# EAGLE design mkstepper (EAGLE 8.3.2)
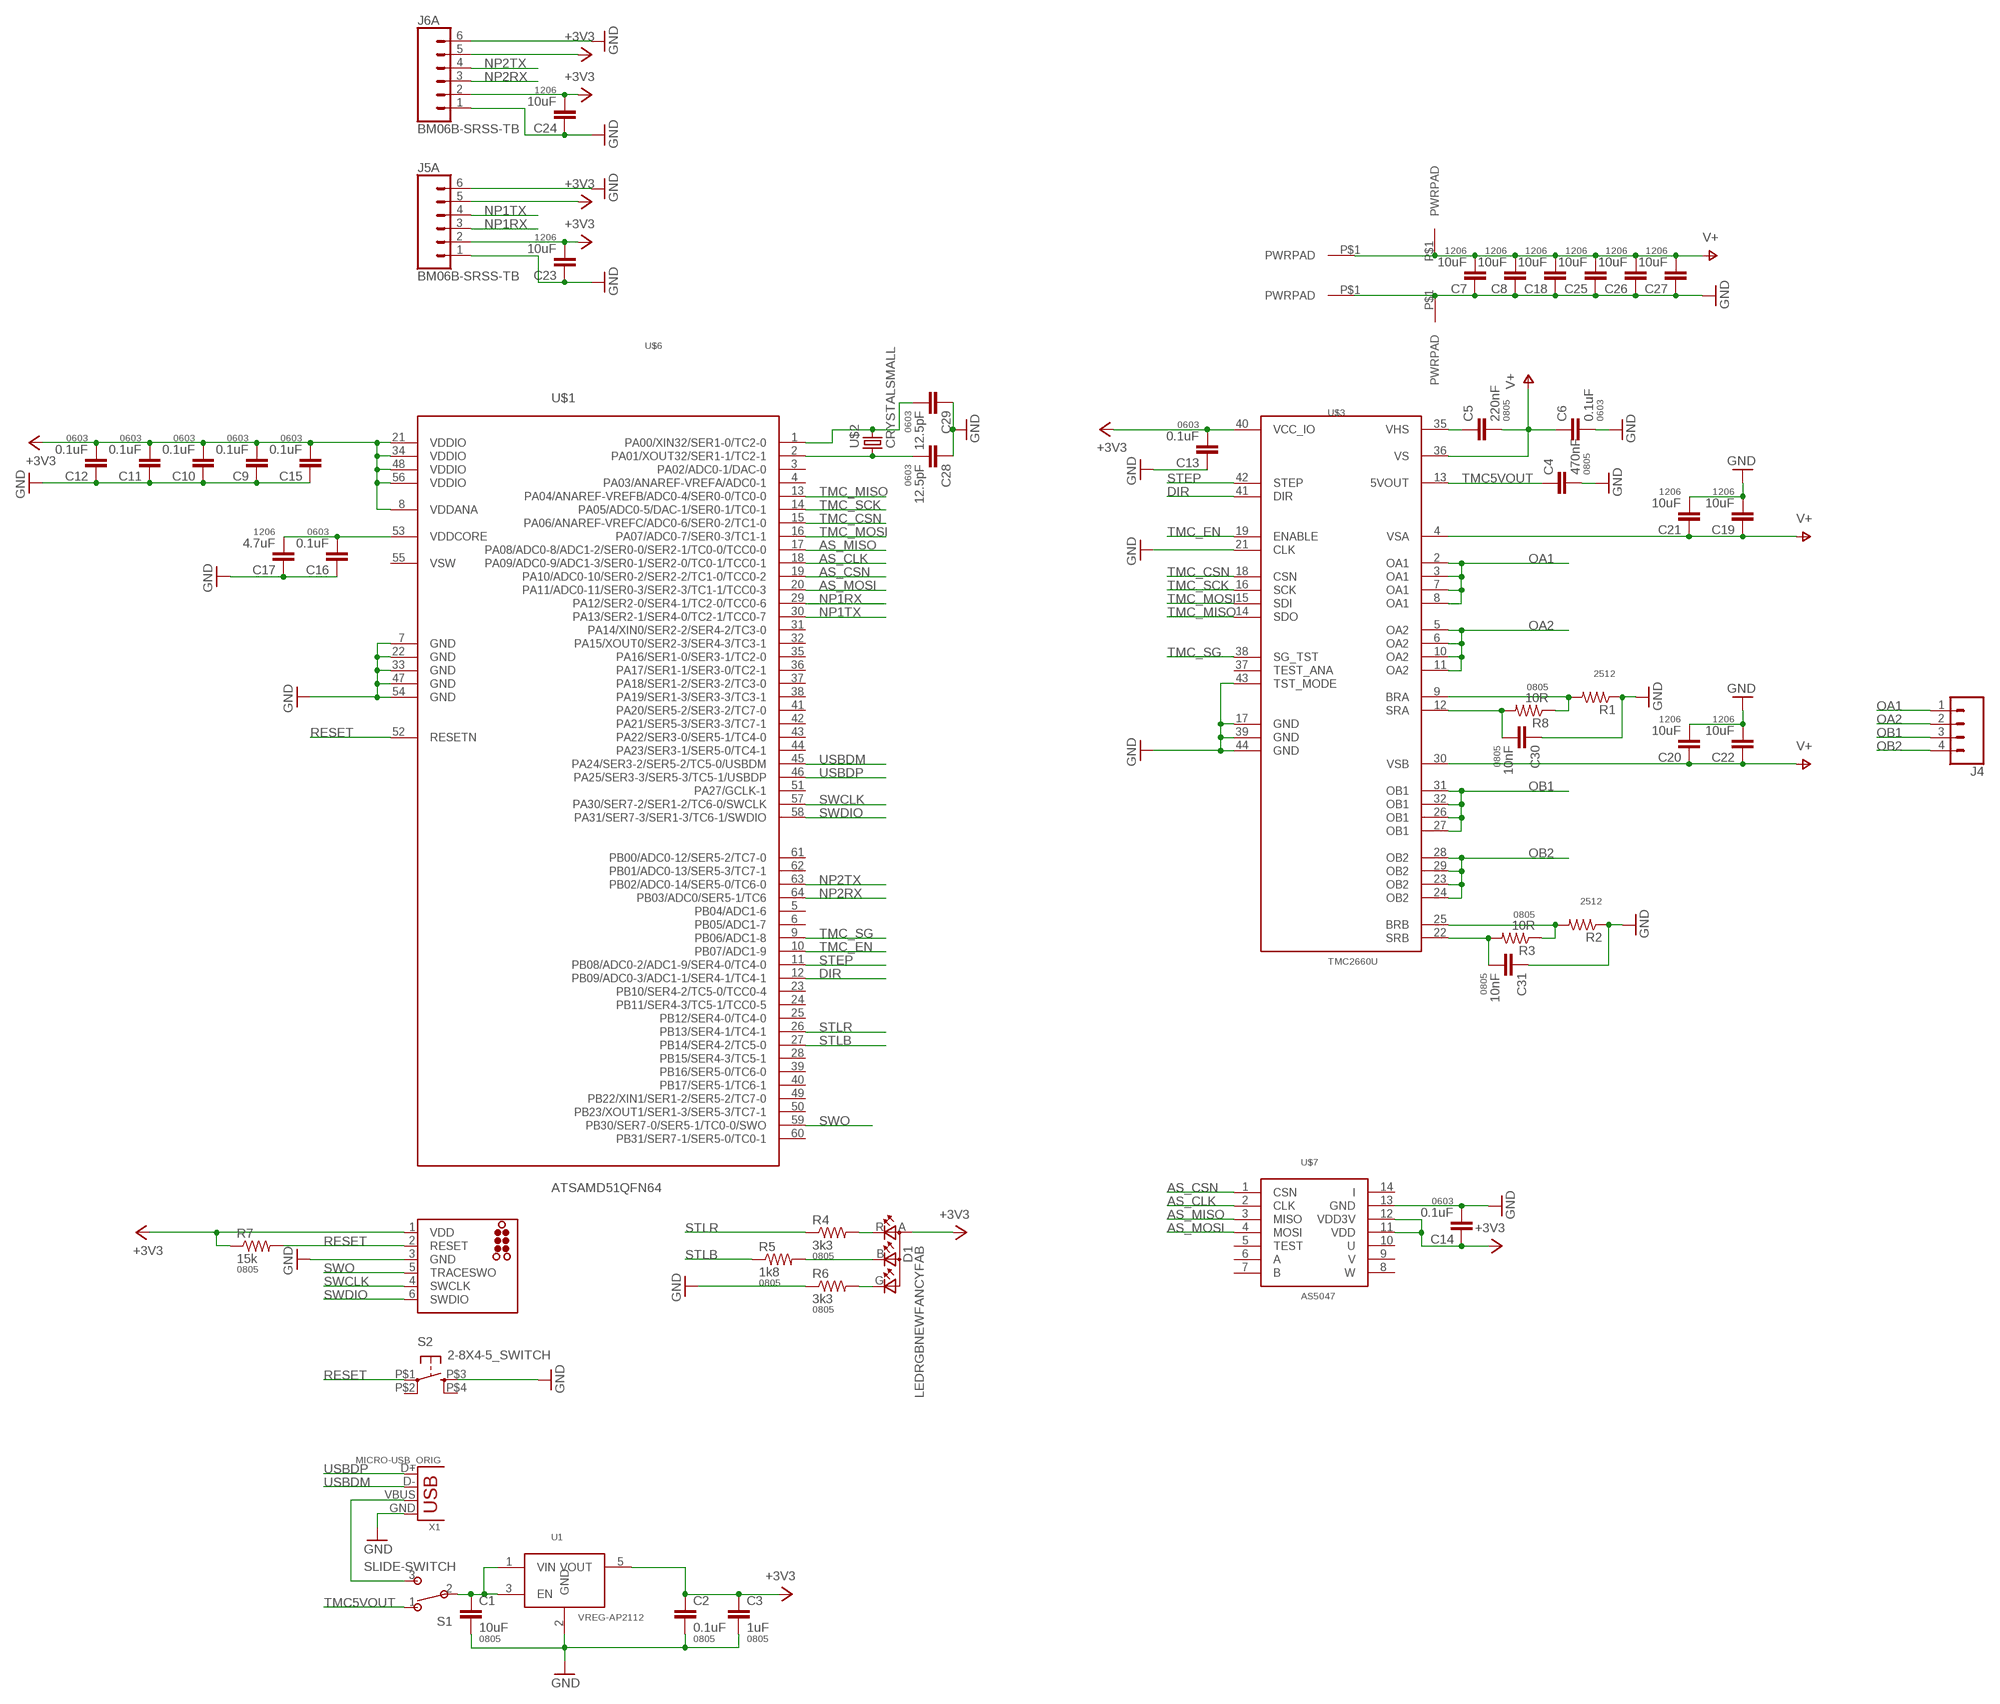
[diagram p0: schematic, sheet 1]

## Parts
C1  10uF  CAP0805  [0805]
C2  0.1uF  CAP0805  [0805]
C3  1uF  CAP0805  [0805]
C4  470nF  CAP0805  [0805]
C5  220nF  CAP0805  [0805]
C6  0.1uF  CAP0603-CAP  [0603-CAP]
C7  10uF  CAP1206  [1206]
C8  10uF  CAP1206  [1206]
C9  0.1uF  CAP0603-CAP  [0603-CAP]
C10  0.1uF  CAP0603-CAP  [0603-CAP]
C11  0.1uF  CAP0603-CAP  [0603-CAP]
C12  0.1uF  CAP0603-CAP  [0603-CAP]
C13  0.1uF  CAP0603-CAP  [0603-CAP]
C14  0.1uF  CAP0603-CAP  [0603-CAP]
C15  0.1uF  CAP0603-CAP  [0603-CAP]
C16  0.1uF  CAP0603-CAP  [0603-CAP]
C17  4.7uF  CAP1206  [1206]
C18  10uF  CAP1206  [1206]
C19  10uF  CAP1206  [1206]
C20  10uF  CAP1206  [1206]
C21  10uF  CAP1206  [1206]
C22  10uF  CAP1206  [1206]
C23  10uF  CAP1206  [1206]
C24  10uF  CAP1206  [1206]
C25  10uF  CAP1206  [1206]
C26  10uF  CAP1206  [1206]
C27  10uF  CAP1206  [1206]
C28  12.5pF  CAP0603-CAP  [0603-CAP]
C29  12.5pF  CAP0603-CAP  [0603-CAP]
C30  10nF  CAP0805  [0805]
C31  10nF  CAP0805  [0805]
D1  LEDRGBNEWFANCYFAB  [P-LCC-4-FANCYFAB]
J1  TC2030-SWD-MCP  [TC2030-MCP]
J2  PWRPADM2  [PWRPAD_2-05MM]
J3  PWRPADM2  [PWRPAD_2-05MM]
J4  CONN_04LONGPADS  [1X04_LONGPADS]
J5  BM06B-SRSS-TB  JST_6_PIN_HORIZONTAL  [JST-6-SMD-HORI-1.0MM]
J6  BM06B-SRSS-TB  JST_6_PIN_HORIZONTAL  [JST-6-SMD-HORI-1.0MM]
J7  PWRPADM2  [PWRPAD_2-05MM]
J9  PWRPADM2  [PWRPAD_2-05MM]
R1  RESISTOR2512  [R2512]
R2  RESISTOR2512  [R2512]
R3  10R  RESISTOR0805-RES  [0805]
R4  3k3  RESISTOR0805-RES  [0805]
R5  1k8  RESISTOR0805-RES  [0805]
R6  3k3  RESISTOR0805-RES  [0805]
R7  15k  RESISTOR0805-RES  [0805]
R8  10R  RESISTOR0805-RES  [0805]
S1  SLIDE-SWITCH  [AYZ0102AGRLC]
S2  2-8X4-5_SWITCH  [TACT-SWITCH-KMR6]
U1  VREG-AP2112  [SOT23-5]
U$1  ATSAMD51QFN64  [QFN-64-9X9MM]
U$2  CRYSTALSMALL  [2-SMD-1-5X3-2MM]
U$3  TMC2660U  [TQFP44]
U$6  NEMA17  [NEMA17]
U$7  AS5047  [TSSOP14]
X1  MICRO-USB_ORIG  [DX4R005HJ5]

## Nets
+3V3: C2.1 C3.1 C9.2 C10.2 C11.2 C12.2 C13.2 C14.1 C15.2 C23.2 C24.2 D1.A(A2) J1.1(VDD) J5.2 J5.5 J6.2 J6.5 R7.1 U1.5(VOUT) U$1.8(VDDANA) U$1.21(VDDIO) U$1.34(VDDIO) U$1.48(VDDIO) U$1.56(VDDIO) U$3.40(VCC_IO) U$7.11(VDD) U$7.12(VDD3V)
AS_CLK: U$1.18(PA09/ADC0-9/ADC1-3/SER0-1/SER2-0/TC0-1/TCC0-1) U$7.2(CLK)
AS_CSN: U$1.19(PA10/ADC0-10/SER0-2/SER2-2/TC1-0/TCC0-2) U$7.1(CSN)
AS_MISO: U$1.17(PA08/ADC0-8/ADC1-2/SER0-0/SER2-1/TC0-0/TCC0-0) U$7.3(MISO)
AS_MOSI: U$1.20(PA11/ADC0-11/SER0-3/SER2-3/TC1-1/TCC0-3) U$7.4(MOSI)
BRA: R1.2 R8.1 U$3.9(BRA)
BRB: R2.2 R3.1 U$3.25(BRB)
DIR: U$1.12(PB09/ADC0-3/ADC1-1/SER4-1/TC4-1) U$3.41(DIR)
GND: C1.2 C2.2 C3.2 C4.2 C6.2 C7.1 C8.1 C9.1 C10.1 C11.1 C12.1 C13.1 C14.2 C15.1 C16.1 C17.1 C18.1 C19.2 C20.2 C21.2 C22.2 C23.1 C24.1 C25.1 C26.1 C27.1 C28.1 C29.1 C30.1 C31.1 J1.3(GND) J3.P$1(PWRPAD) J5.1 J5.6 J6.1 J6.6 J7.P$1(PWRPAD) R1.1 R2.1 R6.1 S2.P$3(S) U1.2(GND) U$1.7(GND) U$1.22(GND) U$1.33(GND) U$1.47(GND) U$1.54(GND) U$3.17(GND) U$3.21(CLK) U$3.39(GND) U$3.43(TST_MODE) U$3.44(GND) U$7.13(GND) X1.GND
N$1: D1.G(CGREEN) R6.2
N$2: C5.1 U$3.35(VHS)
N$3: C1.1 S1.2 U1.1(VIN) U1.3(EN)
N$4: S1.3 X1.VBUS
N$5: D1.B(CBLUE) R5.2
N$6: D1.R(CRED) R4.2
N$7: C16.2 C17.2 U$1.53(VDDCORE)
N$8: C28.2 U$1.2(PA01/XOUT32/SER1-1/TC2-1) U$2.P$1
N$12: C29.2 U$1.1(PA00/XIN32/SER1-0/TC2-0) U$2.P$2
NP1RX: J5.3 U$1.29(PA12/SER2-0/SER4-1/TC2-0/TCC0-6)
NP1TX: J5.4 U$1.30(PA13/SER2-1/SER4-0/TC2-1/TCC0-7)
NP2RX: J6.3 U$1.64(PB03/ADC0/SER5-1/TC6)
NP2TX: J6.4 U$1.63(PB02/ADC0-14/SER5-0/TC6-0)
OA1: J4.1 U$3.2(OA1) U$3.3(OA1) U$3.7(OA1) U$3.8(OA1)
OA2: J4.2 U$3.5(OA2) U$3.6(OA2) U$3.10(OA2) U$3.11(OA2)
OB1: J4.3 U$3.26(OB1) U$3.27(OB1) U$3.31(OB1) U$3.32(OB1)
OB2: J4.4 U$3.23(OB2) U$3.24(OB2) U$3.28(OB2) U$3.29(OB2)
RESET: J1.2(RESET) R7.2 S2.P$1(P) U$1.52(RESETN)
SRA: C30.2 R8.2 U$3.12(SRA)
SRB: C31.2 R3.2 U$3.22(SRB)
STEP: U$1.11(PB08/ADC0-2/ADC1-9/SER4-0/TC4-0) U$3.42(STEP)
STLB: R5.1 U$1.27(PB14/SER4-2/TC5-0)
STLR: R4.1 U$1.26(PB13/SER4-1/TC4-1)
SWCLK: J1.4(SWCLK) U$1.57(PA30/SER7-2/SER1-2/TC6-0/SWCLK)
SWDIO: J1.6(SWDIO) U$1.58(PA31/SER7-3/SER1-3/TC6-1/SWDIO)
SWO: J1.5(TRACESWO) U$1.59(PB30/SER7-0/SER5-1/TC0-0/SWO)
TMC5VOUT: C4.1 S1.1 U$3.13(5VOUT)
TMC_CSN: U$1.15(PA06/ANAREF-VREFC/ADC0-6/SER0-2/TC1-0) U$3.18(CSN)
TMC_EN: U$1.10(PB07/ADC1-9) U$3.19(ENABLE)
TMC_MISO: U$1.13(PA04/ANAREF-VREFB/ADC0-4/SER0-0/TC0-0) U$3.14(SDO)
TMC_MOSI: U$1.16(PA07/ADC0-7/SER0-3/TC1-1) U$3.15(SDI)
TMC_SCK: U$1.14(PA05/ADC0-5/DAC-1/SER0-1/TC0-1) U$3.16(SCK)
TMC_SG: U$1.9(PB06/ADC1-8) U$3.38(SG_TST)
USBDM: U$1.45(PA24/SER3-2/SER5-2/TC5-0/USBDM) X1.D-
USBDP: U$1.46(PA25/SER3-3/SER5-3/TC5-1/USBDP) X1.D+
V+: C5.2 C6.1 C7.2 C8.2 C18.2 C19.1 C20.1 C21.1 C22.1 C25.2 C26.2 C27.2 J2.P$1(PWRPAD) J9.P$1(PWRPAD) U$3.4(VSA) U$3.30(VSB) U$3.36(VS)
Unconnected: J5.M1 J5.M2 J6.M1 J6.M2 S2.P$2(P1) S2.P$4(S1) U$1.3(PA02/ADC0-1/DAC-0) U$1.4(PA03/ANAREF-VREFA/ADC0-1) U$1.5(PB04/ADC1-6) U$1.6(PB05/ADC1-7) U$1.23(PB10/SER4-2/TC5-0/TCC0-4) U$1.24(PB11/SER4-3/TC5-1/TCC0-5) U$1.25(PB12/SER4-0/TC4-0) U$1.28(PB15/SER4-3/TC5-1) U$1.31(PA14/XIN0/SER2-2/SER4-2/TC3-0) U$1.32(PA15/XOUT0/SER2-3/SER4-3/TC3-1) U$1.35(PA16/SER1-0/SER3-1/TC2-0) U$1.36(PA17/SER1-1/SER3-0/TC2-1) U$1.37(PA18/SER1-2/SER3-2/TC3-0) U$1.38(PA19/SER1-3/SER3-3/TC3-1) U$1.39(PB16/SER5-0/TC6-0) U$1.40(PB17/SER5-1/TC6-1) U$1.41(PA20/SER5-2/SER3-2/TC7-0) U$1.42(PA21/SER5-3/SER3-3/TC7-1) U$1.43(PA22/SER3-0/SER5-1/TC4-0) U$1.44(PA23/SER3-1/SER5-0/TC4-1) U$1.49(PB22/XIN1/SER1-2/SER5-2/TC7-0) U$1.50(PB23/XOUT1/SER1-3/SER5-3/TC7-1) U$1.51(PA27/GCLK-1) U$1.55(VSW) U$1.60(PB31/SER7-1/SER5-0/TC0-1) U$1.61(PB00/ADC0-12/SER5-2/TC7-0) U$1.62(PB01/ADC0-13/SER5-3/TC7-1) U$3.37(TEST_ANA) U$7.5(TEST) U$7.6(A) U$7.7(B) U$7.8(W) U$7.9(V) U$7.10(U) U$7.14(I)

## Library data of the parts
C1-C5 C30 C31 = borkedlabs-passives:CAP: Capacitor; PACKAGE: 0805
C6 C9-C16 C28 C29 = borkedlabs-passives:CAP: Capacitor; PACKAGE: 0603
C7 C8 C17-C27 = borkedlabs-passives:CAP: Capacitor; PACKAGE: 1206
D1 = fab:LEDRGBNEW
J1 = atsam:TC2030-SWD: TAG-CONNECT ICSP Connector Manufacturer: Tag-Connect Cable for easy In-Circuit Serial Programming. Designed for Microchip ICD2, suitable for many others. Two variants - one "with legs" (for hands-free fit on PCB) and another "without legs" for quick programming. PADDescription 1MCLR/Vpp 2Vdd 3GND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
J2 J3 J7 J9 = power:PWRPAD
J4 = SparkFun-Connectors:CONN_04: Multi connection point. Often used as Generic Header-pin footprint for 0.1 inch spaced/style header connections On any of the 0.1 inch spaced packages, you can populate with these: Break Away Headers - Straight (PRT-00116) Break Away Male Headers - Right Angle (PRT-00553) Female Headers (PRT-00115)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; PROD_ID: CONN-09696
J5 J6 = SparkFun-Connectors:JST_6_PIN_HORIZONTAL: JST 6 pin horizontal connector JST-SH type. Here is the connector we sell at SparkFun: name (XXX-00000) Datasheet It was used on these SparkFun products: name (XXX-00000) name (XXX-00000); PROD_ID: XXX-00000
R1 R2 = borkedlabs-passives:RESISTOR: Resistor; PACKAGE: 2512
R3-R8 = borkedlabs-passives:RESISTOR: Resistor; PACKAGE: 0805
S1 = fab:SLIDE-SWITCH: SMD slide-switch AYZ0102AGRLC as found in the fablab inventory. Includes the mounting holes. Made by Zaerc.
S2 = fab:2-8X4-5_SWITCH
U1 = power:VREG-AP2112
U$1 = atsam:ATSAMD51
U$2 = fab:CRYSTAL
U$3 = power:TMC2660
U$6 = motors:NEMA17
U$7 = sensor:AS5047
X1 = fab:MICRO-USB: SMD micro USB connector as found in the fablab inventory. Three footprint variants included: original, as described by manufacturer's datasheet for milling with the 1/100" bit for milling with the 1/64" bit Made by Zaerc.

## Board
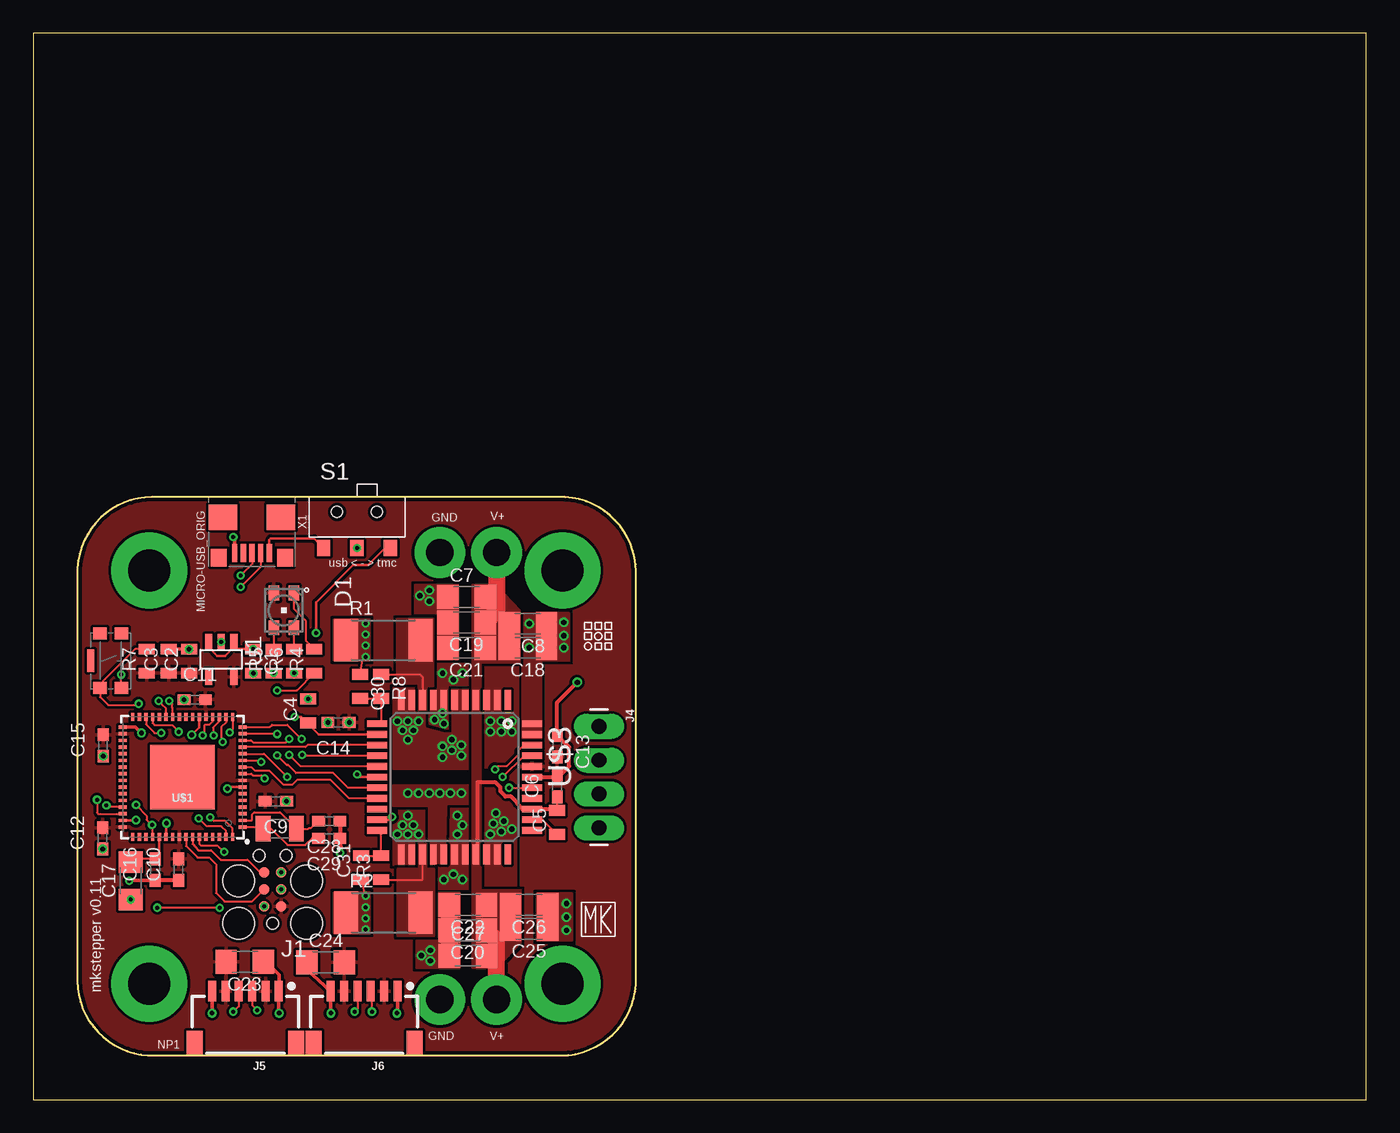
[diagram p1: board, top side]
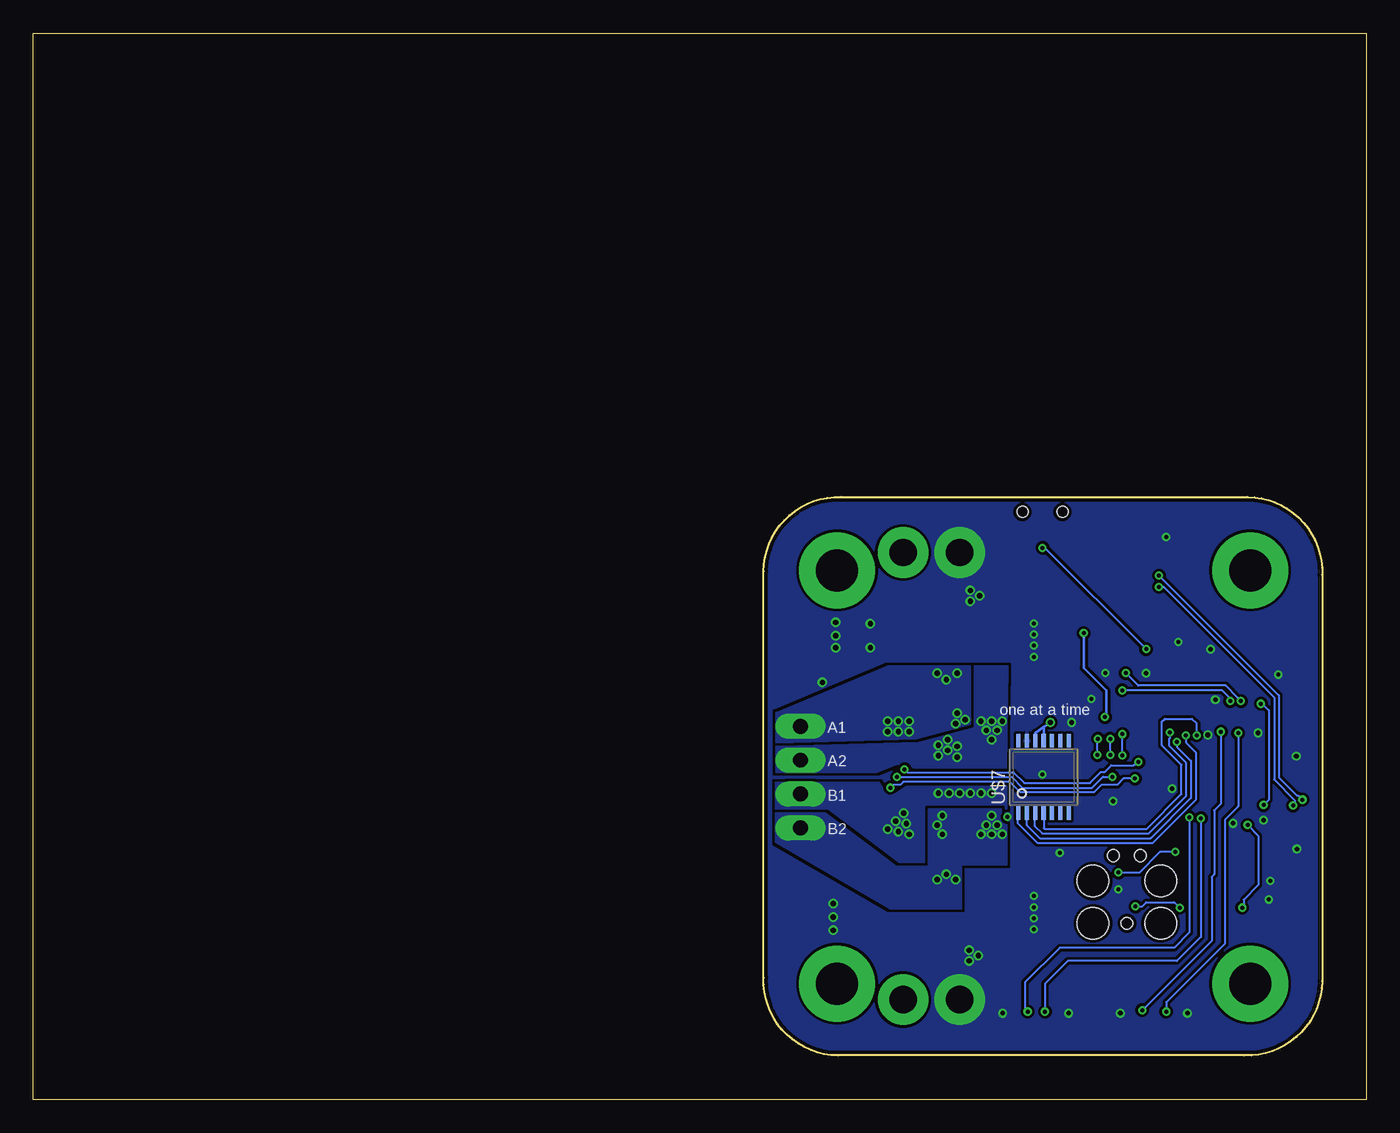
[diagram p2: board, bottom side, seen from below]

Size 100 x 80 mm. Coordinates in mm from the lower left corner, seen from the top.
Outline: 0,0 100,0 100,80 0,80 0,0
Outline: 8.89,45.21 arc91 3.3,39.37 3.3,8.89 arc91 9.14,3.3 39.62,3.3 arc91 45.21,9.14 45.21,39.62 arc91 39.37,45.21 8.89,45.21
Copper layers (1*16): Top 0.035mm / dielectric 1.5mm / Bottom 0.035mm
Design rules "default *": minimum track width 6mil, minimum drill 0.3mm, track to track 8mil, track to pad 8mil, pad to pad 8mil, via to via 8mil, smd to smd 8mil, copper to edge 10mil, drill to drill 10mil, minimum pad ring 6mil, minimum via ring 6mil, stop-mask expansion 4mil, vias tented up to drill 27mil, thermal gap 9mil

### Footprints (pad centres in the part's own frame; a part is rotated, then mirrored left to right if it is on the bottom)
0805 = smd 0.8 x 1.2: 1 -0.9,0; 2 0.9,0
0603-CAP = smd 0.96 x 0.8: 1 -0.8,0; 2 0.8,0
1206 = smd 1.6 x 1.8: 1 -1.4,0; 2 1.4,0
P-LCC-4-FANCYFAB = smd 0.8 x 1.1: A 0.75,-1.3; B 0.75,1.3; G -0.75,1.3; R -0.75,-1.3
TC2030-MCP = smd 0.787 x 0.787: 1 1.27,-0.635; 2 1.27,0.635; 3 2.54,-0.635; 4 2.54,0.635; 5 3.81,-0.635; 6 3.81,0.635 | hole 0.889: 0,0; 5.08,-1.016; 5.08,1.016 | hole 2.375: 0,2.54; 0,-2.54; 3.175,-2.54; 3.175,2.54
PWRPAD_2-05MM = drill 2.05 pad 3.8: P$1 0,0
1X04_LONGPADS = drill 1.118 pad 1.88 long: 1 0,0; 2 2.54,0; 3 5.08,0; 4 7.62,0
JST-6-SMD-HORI-1.0MM = smd 0.6 x 1.55: 1 -2.5,-4.775; 2 -1.5,-4.775; 3 -0.5,-4.775; 4 0.5,-4.775; 5 1.5,-4.775; 6 2.5,-4.775 | smd 1.2 x 1.8: M1 -3.8,-0.9; M2 3.8,-0.9
R2512 = smd 1.8 x 3.2: 1 -2.8,0; 2 2.8,0
AYZ0102AGRLC = smd 1 x 1.2: 1 2.5,-2.3; 2 0,-2.3; 3 -2.5,-2.3 | hole 0.85: -1.5,0.4; 1.5,0.4
TACT-SWITCH-KMR6 = smd 0.9 x 1: P$1 -2.05,0.8; P$2 2.05,0.8; P$3 -2.05,-0.8; P$4 2.05,-0.8 | smd 1.7 x 0.55: P$5 0,1.5
SOT23-5 = smd 0.533 x 1.194: 1 -0.95,-1.306; 2 0,-1.306; 3 0.95,-1.306; 4 0.95,1.306; 5 -0.95,1.306
QFN-64-9X9MM = smd 0.6 x 0.25: 1 -4.5,3.75; 2 -4.5,3.25; 3 -4.5,2.75; 4 -4.5,2.25; 5 -4.5,1.75; 6 -4.5,1.25; 7 -4.5,0.75; 8 -4.5,0.25; 9 -4.5,-0.25; 10 -4.5,-0.75; 11 -4.5,-1.25; 12 -4.5,-1.75; 13 -4.5,-2.25; 14 -4.5,-2.75; 15 -4.5,-3.25; 16 -4.5,-3.75; 33 4.5,-3.75; 34 4.5,-3.25; 35 4.5,-2.75; 36 4.5,-2.25; 37 4.5,-1.75; 38 4.5,-1.25; 39 4.5,-0.75; 40 4.5,-0.25; 41 4.5,0.25; 42 4.5,0.75; 43 4.5,1.25; 44 4.5,1.75; 45 4.5,2.25; 46 4.5,2.75; 47 4.5,3.25; 48 4.5,3.75 | smd 0.25 x 0.6: 17 -3.75,-4.5; 18 -3.25,-4.5; 19 -2.75,-4.5; 20 -2.25,-4.5; 21 -1.75,-4.5; 22 -1.25,-4.5; 23 -0.75,-4.5; 24 -0.25,-4.5; 25 0.25,-4.5; 26 0.75,-4.5; 27 1.25,-4.5; 28 1.75,-4.5; 29 2.25,-4.5; 30 2.75,-4.5; 31 3.25,-4.5; 32 3.75,-4.5; 49 3.75,4.5; 50 3.25,4.5; 51 2.75,4.5; 52 2.25,4.5; 53 1.75,4.5; 54 1.25,4.5; 55 0.75,4.5; 56 0.25,4.5; 57 -0.25,4.5; 58 -0.75,4.5; 59 -1.25,4.5; 60 -1.75,4.5; 61 -2.25,4.5; 62 -2.75,4.5; 63 -3.25,4.5; 64 -3.75,4.5 | smd 4.826 x 4.826: P$1 0,0
2-SMD-1-5X3-2MM = smd 1.1 x 1.9: P$1 -1.25,0; P$2 1.25,0
TQFP44 = smd 1.5 x 0.5: 1 -5.8,4; 2 -5.8,3.2; 3 -5.8,2.4; 4 -5.8,1.6; 5 -5.8,0.8; 6 -5.8,0; 7 -5.8,-0.8; 8 -5.8,-1.6; 9 -5.8,-2.4; 10 -5.8,-3.2; 11 -5.8,-4; 23 5.8,-4; 24 5.8,-3.2; 25 5.8,-2.4; 26 5.8,-1.6; 27 5.8,-0.8; 28 5.8,0; 29 5.8,0.8; 30 5.8,1.6; 31 5.8,2.4; 32 5.8,3.2; 33 5.8,4 | smd 0.5 x 1.5: 12 -4,-5.8; 13 -3.2,-5.8; 14 -2.4,-5.8; 15 -1.6,-5.8; 16 -0.8,-5.8; 17 0,-5.8; 18 0.8,-5.8; 19 1.6,-5.8; 20 2.4,-5.8; 21 3.2,-5.8; 22 4,-5.8; 34 4,5.8; 35 3.2,5.8; 36 2.4,5.8; 37 1.6,5.8; 38 0.8,5.8; 39 0,5.8; 40 -0.8,5.8; 41 -1.6,5.8; 42 -2.4,5.8; 43 -3.2,5.8; 44 -4,5.8
NEMA17 = drill 3.15 pad 5.7: P$1 -15.5,15.5; P$2 15.5,15.5; P$3 -15.5,-15.5; P$4 15.5,-15.5
TSSOP14 = smd 0.305 x 0.991: 1 -1.905,-2.718; 2 -1.27,-2.718; 3 -0.635,-2.718; 4 0,-2.718; 5 0.635,-2.718; 6 1.27,-2.718; 7 1.905,-2.718; 8 1.905,2.718; 9 1.27,2.718; 10 0.635,2.718; 11 0,2.718; 12 -0.635,2.718; 13 -1.27,2.718; 14 -1.905,2.718
DX4R005HJ5 = smd 0.4 x 1.35: D+ 0,1.6; D- -0.65,1.6; GND 1.3,1.6; ID 0.65,1.6; VBUS -1.3,1.6 | smd 1.2 x 1.3: GND@1 -2.5,1.95; GND@2 2.5,1.95 | smd 2.15 x 1.9: GND@3 -2.175,-1.1; GND@4 2.175,-1.1

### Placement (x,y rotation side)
C1  16.51,32.89 270 top
C2  11.68,32.89 90 top
C3  10.16,32.89 90 top
C4  20.61,29.16 90 top
C5  39.3,20.8 90 top
C6  39.3,23.5 90 top
C7  32.5,37.7 0 top
C8  37.1,35.7 180 top
C9  18.2,22.38 180 top
C10  10.9,17.25 90 top
C11  12.11,30 0 top
C12  5.2,19.6 90 top
C13  39.3,26.5 270 top
C14  22.9,28.3 180 top
C15  5.24,26.57 90 top
C16  9.15,17.25 90 top
C17  7.3,16.4 90 top
C18  37.1,33.9 180 top
C19  32.5,35.8 180 top
C20  32.6,12.7 180 top
C21  32.5,33.9 180 top
C22  32.6,14.6 180 top
C23  15.87,10.32 180 top
C24  21.93,10.3 0 top
C25  37.2,12.8 180 top
C26  37.2,14.6 180 top
C27  32.6,10.8 0 top
C28  22.2,20.9 180 top
C29  22.2,19.6 180 top
C30  24.5,31 270 top
C31  24.6,17.4 90 top
D1  18.8,36.7 180 top
J1  17.95,13.22 90 top
J2  34.75,41.04 0 top
J3  30.5,41.04 0 top
J4  42.45,28 270 top
J5  15.92,3.35 180 top
J6  24.82,3.35 180 top
J7  30.5,7.5 0 top
J9  34.75,7.5 0 top
R1  26.26,34.47 0 top
R2  26.27,14.01 0 top
R3  26.1,17.4 90 top
R4  21.08,32.89 90 top
R5  18.03,32.89 90 top
R6  19.56,32.89 90 top
R7  8.51,32.89 90 top
R8  26.1,31 270 top
S1  24.28,43.69 0 top
S2  5.81,32.92 90 top
U1  14.1,33.02 180 top
U$1  11.2,24.2 180 top
U$2  18.49,20.32 180 top
U$3  31.6,24.2 270 top
U$5  [CBA-SILK-LOGO]  42.38,34.77 90 top
U$6  24.2,24.2 0 top
U$7  24.2,24.2 0 bottom
U$9  [MK-LOGO-SILK]  42.38,13.51 0 top
X1  16.4,42.6 180 top

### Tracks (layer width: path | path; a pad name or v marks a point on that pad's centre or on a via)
+3V3  (via drill 0.35)
  Bottom 0.2: C14.1 23.9,28.15 24.13,28 | U$7.12 24.84,27.52 24.13,28 | U$7.11 24.2,27.92 24.13,28
  other vias: 23.7,28.3
  pour Top (rank 6): 3.15,39.65 3.3,45.21 8.7,45.2 39.7,45.2 45.21,45.21 45.25,39.65 45.25,8.7 45.21,3.3 39.7,3.15 8.7,3.15 3.3,3.3 3.15,8.7
AS_CLK  (via drill 0.3 pad 0.42)
  Top 0.152: U$1.18 14.45,28.29 14.1,27.94 14.1,27.56 14.11,27.55 14.11,26.91 v14.19,26.83
  Bottom 0.152: U$7.2 25.45,21.46 25.45,20.57 24.49,19.61 16.16,19.61 13.14,22.63 13.14,25.41 14.19,26.46 v14.19,26.83
AS_CSN  (via drill 0.3 pad 0.42)
  Top 0.152: U$1.19 13.95,28.38 13.49,27.91 13.49,27.35 v13.53,27.3
  Bottom 0.152: U$7.1 26.14,21.45 26.14,20.73 24.66,19.25 16.01,19.25 12.79,22.48 12.79,26.05 13.53,26.79 v13.53,27.3
AS_MISO  (via drill 0.3 pad 0.42)
  Top 0.152: U$1.17 14.95,27.78 v14.73,27.56
  Bottom 0.152: U$7.3 24.84,20.5 24.31,19.96 16.31,19.96 13.5,22.77 13.5,25.26 14.78,26.54 14.78,27.07 14.73,27.11 v14.73,27.56
AS_MOSI  (via drill 0.3 pad 0.42)
  Top 0.152: U$1.20 13.45,28.38 13.19,28.12 12.88,28.12 12.83,28.07 12.83,27.44 v12.72,27.33
  Bottom 0.152: U$7.4 24.2,20.36 24.16,20.32 16.45,20.32 13.85,22.92 13.85,25.12 15.31,26.58 15.31,28.37 15.11,28.57 13.08,28.57 12.72,28.21 v12.72,27.33
BRA
  Top 0.152: R8.1 29,31.9 29.2,31.7 U$3.9
  pour Top (no thermals): 28.9,29.2 28.9,31.2 27.3,31.2 27.3,36.1 30,36.1 30,31 29.5,31 29.5,29.2
BRB
  Top 0.152: R3.1 29.2,16.5 U$3.25
  pour Top (no thermals): 28.9,19.2 28.9,17.3 27.3,17.3 27.3,12.3 30.1,12.3 30.1,17.3 29.5,17.3 29.5,19.2
DIR  (via drill 0.3, 0.3 pad 0.42)
  Top 0.152: U$1.12 17.31,25.95 v19.04,24.22 | U$3.41 36.8,25.8 v35.2,24.2
  Top 0.2: 36.77,25.8 U$3.41
  Bottom 0.152: v35.2,24.2 26.6,24.2 25.8,23.4 20.57,23.4 19.75,24.22 v19.04,24.22 | v19.04,24.22
GND  (via drill 0.3, 0.3 pad 0.42, 0.35, 0.4 pad 0.42)
  Top 0.152: S2.P$3 v6.61,31.87 v6.6,31.88 | v24.94,15.27 25,15.33 24.8,15.53 C31.1 | 25,33.16 v24.94,33.22 24.7,32.98 C30.1
  Top 0.2: U$3.17 24.5,24.2 v24.3,24.4 | U$3.21 26.71,21 v26.91,21.19 | 39.25,27.4 C13.1 | 39.2,24.3 C6.2
  Top 0.203: 9.09,16.34 C16.1 | U$1.54 9.95,20.69 v9.98,20.73 | U$1.47 v7.69,20.95 v7.7,20.95 | U$1.7 14.69,23.45 v14.55,23.32 | U$1.22 12.45,27.92 v11.89,27.36
  Top 0.254: X1.GND 15.1,42.13 v15.01,42.22 | U$1.33 7.66,27.95 v8.1,27.51 | C3.2 C2.2 | v18.44,6.48 18.42,6.49 J5.1 18.44,7.94 18.44,9.37 17.59,10.22 C23.1 | J5.6 13.42,6.49 v13.41,6.48 | v22.33,6.48 22.32,6.49 J6.6 20.53,9.72 C24.1 | J6.1 27.32,6.52 v27.28,6.48
  Top 0.305: C28.1 C29.1 23.05,18.55 v23,18.5 | C6.2 39.6,24.4 40.16,24.95 40.16,24.96 40.2,25 40.2,26.45 C13.1 39.3,29.8 v40.8,31.3 | U$3.39 39.1,24.2 39.2,24.3 | C10.1 C16.1 v7.2,16.4
  Top 1.27: C22.2 C20.2 C27.1 | C18.1 C8.1 | C25.1 C26.1
  other vias: 22.1,28.3 24.94,35.73 24.94,34.06 24.94,34.9 24.94,12.75 24.94,13.59 24.94,14.43 7.3,15 5.24,25.77 11.31,30 19,22.38 16.51,31.99 11.68,33.79 5.2,18.8 14.1,34.33 18.59,15.76 19.56,31.99 20.61,30.06 40,14.7 40,13.7 40,12.7 29.8,11.2 29.8,10.4 29.1,10.8 39.8,35.8 39.8,34.8 39.8,33.9 29.7,38.2 29.7,37.4 29,37.8 37.2,33.9 37.2,35.7
  pour Bottom (rank 4): 3.15,39.65 3.3,45.21 8.7,45.2 39.7,45.2 45.21,45.21 45.25,39.65 45.25,8.7 45.21,3.3 39.7,3.15 8.7,3.15 3.3,3.3 3.15,8.7
  pour Top (no thermals): 22.57,36.04 25.24,36.04 25.24,32.91 22.57,32.91
  pour Top (no thermals): 22.57,15.57 25.24,15.57 25.24,12.45 22.57,12.45
  pour Top (no thermals): 37.8,15.5 40.4,15.5 40.4,11.9 37.8,11.9
  pour Top (rank 3, no thermals): 32,9.9 32,15.5 30.4,15.5 30.4,11.9 28.7,11.9 28.7,9.9
  pour Top (no thermals): 37.7,36.5 37.7,33 40.2,33 40.2,36.5
  pour Top (rank 3, no thermals): 30.3,33 31.9,33 31.9,38.6 28.6,38.6 28.6,36.5 30.3,36.5
  pour Top (rank 2, no thermals): 36.7,27.1 36.7,36.5 40.2,36.5 40.2,32.9 38.1,32.9 38.1,27.1
N$1
  Top 0.152: D1.G 19.55,33.8 R6.2
N$2
  Top 0.2: U$3.35 38.2,21 C5.1
N$3  (via drill 0.3 pad 0.42)
  Top 0.2: U1.3 13.15,33.95 13.8,33.3 14.4,33.3 15.05,33.95 15.05,34 | 15.05,34 U1.1 | C1.1 15.25,33.79 15.05,34
  Bottom 0.2: S1.2 24.11,41.39 C1.1
  other vias: 16.51,33.79 24.28,41.39
N$4
  Top 0.2: X1.VBUS 17.7,42 17.8,42.1 21.07,42.1 S1.3
N$5
  Top 0.152: D1.B 18.05,33.8 R5.2
N$6
  Top 0.152: D1.R 19.55,36.84 20.45,35.94 20.45,34.43 R4.2
N$7
  Top 0.203: U$1.53 9.45,18.4 C16.2 7.6,18.1 C17.2
N$8
  Top 0.152: U$1.2 16.41,20.95 16.41,21.39 16.57,21.55 18.51,21.55 U$2.P$1 20.62,20.32 20.68,20.38 20.83,20.38 C28.2
N$12
  Top 0.152: U$1.1 16.91,20.45 U$2.P$2 17.84,20.32 19.07,19.09 20.4,19.09 20.91,19.6 C29.2
NP1RX  (via drill 0.3 pad 0.42)
  Top 0.152: U$1.29 8.95,28.25 9.1,28.1 10.4,28.1 v10.9,27.6 | J5.3 16.42,7.08 v16.8,6.7
  Bottom 0.152: v10.9,27.6 10.9,22.2 11.4,21.7 11.4,16.9 11.6,16.7 11.6,11.9 v16.8,6.7
NP1TX  (via drill 0.3 pad 0.42)
  Top 0.152: U$1.30 8.45,28.15 9.1,27.5 v9.6,27.5 | J5.4 15.42,6.98 v15,6.6
  Bottom 0.152: v9.6,27.5 9.6,22 10.6,21 10.6,11.7 15,7.3 v15,6.6
NP2RX  (via drill 0.3 pad 0.42)
  Top 0.152: U$1.64 14.95,20.35 14.4,20.9 13.54,20.9 v13.27,21.17 | v25.4,6.6 25.4,8.05 J6.3
  Bottom 0.152: v13.27,21.17 13.27,12.53 14.4,11.4 23,11.4 25.6,8.8 25.6,6.8 v25.4,6.6
NP2TX  (via drill 0.3 pad 0.42)
  Top 0.152: U$1.63 14.45,20.15 14.1,20.5 13,20.5 v12.4,21.1 | J6.4 24.32,6.82 v24.1,6.6
  Bottom 0.152: v12.4,21.1 12.4,12.2 14.2,10.4 22.4,10.4 24.1,8.7 v24.1,6.6
OA1  (via drill 0.4 pad 0.42)
  other vias: 30.7,29 30.8,28.2 30.1,28.5 34.3,27.6 35.1,27.6 35.9,27.6 30.7,32 32.2,32 31.5,31.5 34.3,28.4 35.1,28.4 35.9,28.4
  pour Bottom (rank 2, no thermals): 44.3,26.8 33.8,27.1 29.7,28.2 29.7,32.5 35.9,32.5 44.2,29 44.3,29
  pour Top (rank 2, no thermals): 30.2,32.7 30.2,30.9 29.7,30.9 29.7,28.2 31.1,27.8 31.1,31.1 32.8,31.1 32.8,32.7
  pour Top (rank 2, no thermals): 33.6,32.7 33.6,27.2 33.7,24.9 36.4,25 36.4,32.7
OA2  (via drill 0.4 pad 0.42)
  other vias: 28.5,27.7 28.1,28.4 28.9,28.4 27.7,27.7 27.3,28.4 28.1,27 31.4,27 31.4,26.2 32.1,26.6 32.1,25.8 30.7,26.5 30.7,25.7
  pour Bottom (rank 3, no thermals): 44.3,24.6 36.7,24.6 35.2,25.2 34.3,25.2 33.8,24.8 27,24.8 26.9,32.5 29.4,32.5 29.5,28 33.9,26.9 44.3,26.5
  pour Top (rank 3, no thermals): 28.8,30.9 27,30.9 27,24.8 33.8,24.8 34.3,25.2 35.4,25.2 36.2,26 36.2,26.8 34.3,26.8 33.5,27 33.5,29.1 32.8,29.1 32.8,30.8 31.3,30.8 31.3,27.6 29.5,28.1 29.5,29.1 28.8,29.1
OB1  (via drill 0.4 pad 0.42)
  other vias: 29.7,23 28.9,23 28.1,23 30.5,23 31.3,23 32.1,23 34.3,19.9 35.1,20.1 34.7,21.5 35.9,20.3 35.3,20.9 34.5,20.7
  pour Bottom (rank 2, no thermals): 44.3,23.8 36.6,23.8 36.1,23 36,22.9 35.4,22.9 34.3,23.6 27,23.6 27,21.8 32.9,21.8 32.9,17.7 35.2,17.7 36.3,18.6 40.8,21.8 44.3,21.8
  pour Top (rank 4, no thermals): 29.7,17.6 29.7,22 27,22 27,23.6 34.3,23.6 35.4,22.9 36.2,22.9 36.2,15.8 33.6,15.8 33.6,19.4 32.9,19.4 33,21.8 31.2,21.8 31.1,17.6
OB2  (via drill 0.4 pad 0.42)
  other vias: 28.1,19.9 27.3,19.9 28.9,19.9 27.7,20.6 28.5,20.6 28.1,21.3 31.8,19.9 32.2,20.6 31.8,21.3 31.5,16.9 32.2,16.5 30.8,16.5
  pour Bottom (no thermals): 44.3,21.5 40.6,21.5 37,18.8 35.3,17.5 32.8,17.5 32.8,21.8 27.4,21.8 27.4,20.9 27,20.7 27,17.6 30.4,17.6 30.4,14.3 35.7,14.3 44.3,19.3
  pour Top (rank 5, no thermals): 28.7,17.6 28.7,19.3 29.6,19.3 29.6,21.8 27.4,21.8 27.4,20.9 27,20.7 27,17.6
  pour Top (rank 3, no thermals): 31.3,21.8 31.2,17.5 30.2,17.5 30.2,15.8 32.8,15.8 32.9,21.8
RESET  (via drill 0.3 pad 0.42)
  Top 0.152: R7.2 7.63,33.79 5.21,31.37 5.21,31.07 S2.P$1 5.01,30.19 5.6,29.6 7.8,29.6 v7.9,29.7 | v13.99,14.39 9.41,14.39 v9.3,14.4 | U$1.52 8.95,20.55 v8.9,20.6 8.5,21 8.5,21.3 v7.7,22.1
  Bottom 0.152: J1.2 16.81,14.49 16.5,14.8 14.4,14.8 v13.99,14.39 | v8.9,20.6 8.1,19.8 8.1,16.1 9.2,15 9.2,14.5 v9.3,14.4 | v7.9,29.7 7.8,29.7 7.3,29.2 7.3,22.5 v7.7,22.1
  other vias: 17.32,14.49
SRA
  Top 0.152: C30.2 R8.2 26.1,28.5 U$3.12
SRB
  Top 0.152: C31.2 R3.2 26.1,19.9 U$3.22
STEP  (via drill 0.3, 0.3 pad 0.42)
  Top 0.152: U$1.11 16.95,25.45 v17.09,25.32 | 36.78,26.6 U$3.42 36.8,26.6 36.37,26.17 36.37,25.87 35.5,25 34.86,25 v34.64,24.78
  Bottom 0.152: v17.09,25.32 17.2,25.32 17.45,25.07 19.13,25.07 19.62,24.58 19.89,24.58 20.71,23.76 25.65,23.76 26.45,24.56 34.4,24.56 34.63,24.78 v34.64,24.78
STLB  (via drill 0.3 pad 0.42)
  Top 0.152: U$1.27 9.95,29.33 9.62,29.66 9.62,29.67 v9.39,29.9
  Bottom 0.152: v9.39,29.9 9.62,30.13 9.62,30.14 10.53,31.06 17.1,31.06 R5.1
  other vias: 18.03,31.99
STLR  (via drill 0.3 pad 0.42)
  Top 0.152: U$1.26 10.45,29.37 10.43,29.39 10.43,29.67 v10.2,29.9 | v18.3,30.7 19.79,30.7 R4.1
  Bottom 0.152: v10.2,29.9 10.2,30.1 10.8,30.7 v18.3,30.7
SWCLK
  Top 0.152: U$1.57 11.45,19.03 12.32,18.16 13.21,18.16 13.72,17.65 13.72,15.49 14.35,14.86 16.41,14.86 J1.4
SWDIO
  Top 0.152: J1.6 17.03,17.03 16.08,17.98 14.06,17.98 13.34,18.7 12.37,18.7 11.95,19.17 U$1.58
SWO  (via drill 0.3 pad 0.42)
  Top 0.152: U$1.59 12.45,19.2 12.57,19.06 13.81,19.06 v14.3,18.57
  Bottom 0.152: v14.3,18.57 15.47,18.57 17.02,17.02 18.57,17.02 J1.5
  other vias: 18.59,17.03
TMC5VOUT  (via drill 0.3 pad 0.42)
  Top 0.2: U$3.13 21.4,27.4 20.61,28.19 20.61,28.2 | 20.61,28.2 C4.1 | S1.1 26.39,41.39 25.1,40.1 24,40.1 21.2,37.3 v21.2,35 | v19.6,28.7 20.11,28.7 20.61,28.2
  Bottom 0.2: v21.2,35 21.2,32.4 19.5,30.7 19.5,28.8 v19.6,28.7
TMC_CSN  (via drill 0.3)
  Top 0.152: v18.29,27.41 15.74,27.41 U$1.15 | U$3.18 23.6,23.4 22.5,24.5 19.7,24.5 19.1,25.1 19.02,25.1 v18.29,25.83
  Bottom 0.152: v18.29,25.83 v18.29,27.41
TMC_EN
  Top 0.152: U$1.10 16.35,24.95 16.61,24.69 17.71,24.69 18.79,23.61 19.42,23.61 19.81,24 22.3,24 23.7,22.6 U$3.19
TMC_MISO
  Top 0.152: U$1.13 20.41,26.45 20.56,26.6 U$3.14
TMC_MOSI  (via drill 0.3)
  Top 0.152: v20.12,27.06 v20.11,27.06 19.05,28.12 17.91,28.12 17.74,27.95 U$1.16 | U$3.15 20.2,25.8 v20.16,25.84
  Bottom 0.152: v20.16,25.84 20.16,27.01 v20.12,27.06
TMC_SCK  (via drill 0.3)
  Top 0.152: U$1.14 16.33,26.95 16.48,26.81 18.95,26.81 v19.2,27.06 | v19.2,25.84 20.05,25 U$3.16
  Bottom 0.152: v19.2,25.84 v19.2,27.06
TMC_SG  (via drill 0.3, 0.3 pad 0.42)
  Top 0.152: U$1.9 16.35,24.45 16.46,24.33 17.1,24.33 v17.35,24.08 | v35.7,23.4 U$3.38
  Bottom 0.152: v17.35,24.08 18.21,24.08 18.68,23.61 19.85,23.61 20.42,23.04 25.95,23.04 26.75,23.84 34.73,23.84 34.96,23.62 35.48,23.62 v35.7,23.4
USBDM  (via drill 0.3)
  Top 0.152: X1.D- 17.05,39.97 v15.54,38.46 | U$1.45 5.59,21.95 v5.49,22.06
  Bottom 0.152: v15.54,38.46 15.19,38.46 6.91,30.18 6.91,24.01 5.36,22.46 5.36,22.19 v5.49,22.06
USBDP  (via drill 0.3, 0.3 pad 0.42)
  Top 0.152: X1.D+ 16.4,40.17 v15.54,39.32 | U$1.46 4.84,21.45 4.78,21.51 v4.78,22.5
  Bottom 0.152: v15.54,39.32 6.55,30.33 6.55,24.16 5.2,22.8 5.08,22.8 v4.78,22.5
V+
  Top 0.2: C5.2 C6.1
  Top 0.305: U$3.30 33.3,18.5 33.3,23.8 33.31,23.79 34.69,23.79 35.04,23.43 35.04,23.13 35.43,22.74 35.86,22.74 36.29,22.31 36.29,22.2 36.7,21.8 U$3.36 39.2,21.8 C5.2
  Top 1.27: J9.P$1 34.75,11.95 C20.1 | J2.P$1 34.75,36.65 C19.1
  pour Top (no thermals): 36.5,36.7 34.7,38.6 33.1,38.6 32.9,38.6 32.9,9.9 34.8,9.9 36.6,11.8 36.6,15.5 36.6,15.7 33.6,15.7 33.6,32.8 36.5,32.8

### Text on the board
tPlace: GND | V+ | usb < - > tmc | mkstepper v0.11 | NP1 | GND | V+
bPlace: one at a time | A1 | A2 | B1 | B2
